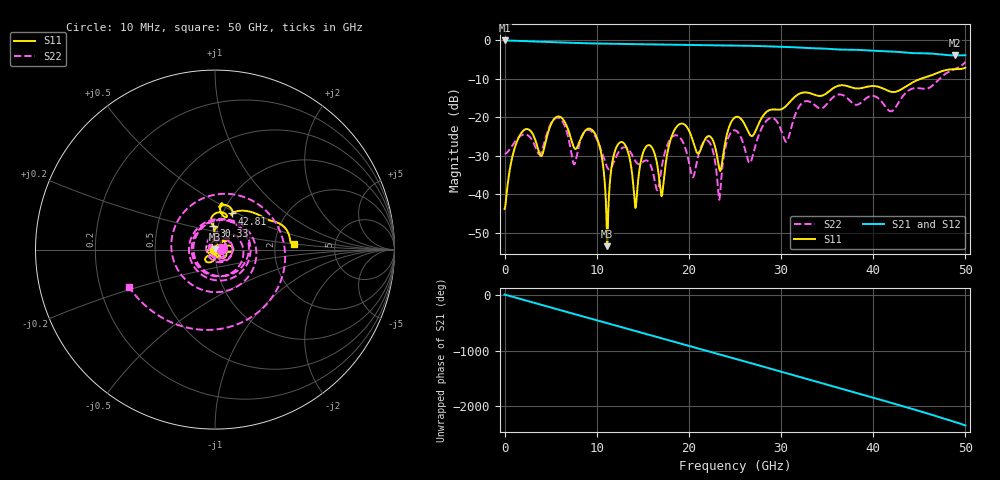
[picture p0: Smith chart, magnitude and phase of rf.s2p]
!  2-Port S-parameters saved by WinCal
! VAR NAME=rf_2
! VAR DATE=11/6/2018 3:01:48 PM
! VAR FILENAME=rf_2_1.S2P
# Hz S DB R 50
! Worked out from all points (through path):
!   5000 points, 10 MHz to 50 GHz, reference 50 ohm
!   highest |S21| = -0.01 dB at 10 MHz (marker M1); lowest = -3.9 dB at 48.87 GHz (marker M2)
!   group delay of S21, straight-line fit = 129 ps
!   lowest |S11| = -53.5 dB at 11.15 GHz (marker M3), VSWR 1.00, Z = 50.1 + j0.199 ohm
!   |S11| at or under -10 dB: start of sweep to 45.13 GHz
!   |S22| runs from -41.5 to -5.6 dB; largest |S21 - S12| = 0
!   S11 on the Smith chart (normalised r, x): 10 MHz: 0.99, +0.00; 30.33 GHz: 0.95, +0.26; 42.81 GHz: 1.11, +0.47; 50 GHz: 2.56, +0.21
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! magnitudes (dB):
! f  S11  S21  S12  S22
! 10 MHz  -43.8  0.0  0.0  -29.5
! 2.05 GHz  -23.5  -0.2  -0.2  -24.5
! 8.35 GHz  -25.1  -0.7  -0.7  -25.3
! 10.09 GHz  -25.8  -0.8  -0.8  -26.1
! 11.15 GHz  -53.5  -0.9  -0.9  -33.1
! 12.48 GHz  -26.6  -0.9  -0.9  -28.7
! 14.19 GHz  -43.5  -1.0  -1.0  -31.4
! 15.4 GHz  -27.5  -1.0  -1.0  -31.2
! 16.68 GHz  -34.1  -1.0  -1.0  -38.5
! 18.6 GHz  -22.7  -1.1  -1.1  -24.7
! 20.42 GHz  -26.0  -1.2  -1.2  -35.6
! 22.19 GHz  -24.9  -1.2  -1.2  -26.4
! 23.31 GHz  -33.5  -1.3  -1.3  -41.4
! 25.01 GHz  -20.0  -1.3  -1.3  -23.4
! 26.59 GHz  -24.4  -1.4  -1.4  -31.9
! 28.63 GHz  -18.3  -1.5  -1.5  -20.5
! 30.33 GHz  -17.5  -1.7  -1.7  -25.5
! 33.34 GHz  -13.9  -2.0  -2.0  -16.3
! 41.67 GHz  -13.2  -2.8  -2.8  -18.2
! 42.81 GHz  -13.0  -3.0  -3.0  -15.9
! 48.87 GHz  -7.5  -3.9  -3.9  -7.4
! 50 GHz  -7.1  -3.9  -3.9  -5.6
